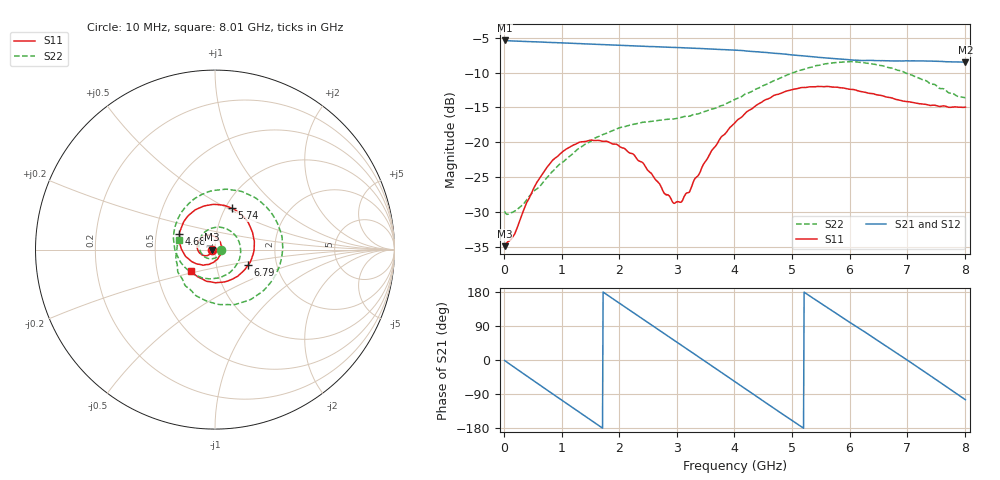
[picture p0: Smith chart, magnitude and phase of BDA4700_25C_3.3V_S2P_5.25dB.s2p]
!Agilent Technologies,E5071B,MY42404982,A.09.10
!Date: Mon Oct 20 18:05:11 2025
!Data & Calibration Information:
!Freq	S11:SOLT2(ON)	S21:SOLT2(ON)	S12:SOLT2(ON)	S22:SOLT2(ON)
# Hz S RI R 50
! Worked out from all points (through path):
!   801 points, 10 MHz to 8.01 GHz, reference 50 ohm
!   highest |S21| = -5.37 dB at 10 MHz (marker M1); lowest = -8.5 dB at 8.01 GHz (marker M2)
!   group delay of S21, straight-line fit = 285 ps
!   lowest |S11| = -34.9 dB at 10 MHz (marker M3), VSWR 1.04, Z = 48.2 - j0.11 ohm
!   |S11| at or under -10 dB: start of sweep to end of sweep
!   |S22| runs from -30.4 to -8.4 dB; largest |S21 - S12| = 0.0063
!   S11 on the Smith chart (normalised r, x): 10 MHz: 0.96, -0.00; 4.68 GHz: 0.66, +0.12; 5.74 GHz: 1.07, +0.53; 6.79 GHz: 1.43, -0.26; 8.01 GHz: 0.74, -0.18
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1e7  -0.0179 -0.00113  0.5387 -0.0118  0.5388 -0.0121  0.0317 -0.00258
3.3e8  -0.0239 -0.0207  0.4328 -0.307  0.4325 -0.3072  0.0222 -0.028
7.1e8  -0.0526 -0.0343  0.1322 -0.5064  0.1321 -0.5064  -0.0163 -0.0511
1.02e9  -0.0831 -0.0214  -0.1581 -0.4922  -0.1584 -0.4926  -0.0622 -0.0363
1.35e9  -0.0998 0.0138  -0.4038 -0.3121  -0.4041 -0.3124  -0.0901 0.0229
1.93e9  -0.06 0.0762  -0.4601 0.1917  -0.4603 0.1914  -0.00232 0.123
2.32e9  -0.0081 0.0741  -0.224 0.4365  -0.224 0.4368  0.1007 0.0921
2.68e9  0.0292 0.0422  0.0838 0.4775  0.0832 0.4774  0.1433 -0.00884
3.05e9  0.0351 -0.0118  0.3569 0.3184  0.3538 0.3208  0.0964 -0.1144
3.36e9  0.0103 -0.0561  0.4653 0.0819  0.4659 0.0821  0.00735 -0.1593
3.67e9  -0.0425 -0.0831  0.432 -0.1749  0.432 -0.1764  -0.0969 -0.1466
4.01e9  -0.1175 -0.0729  0.2476 -0.3864  0.2483 -0.3856  -0.19 -0.0718
4.34e9  -0.1783 -0.0129  -0.0116 -0.4479  -0.0116 -0.4486  -0.2307 0.0516
4.68e9  -0.1984 0.0869  -0.2609 -0.3491  -0.2599 -0.3507  -0.1949 0.1957
5.02e9  -0.1509 0.1866  -0.4013 -0.134  -0.4026 -0.1346  -0.0706 0.3087
5.35e9  -0.0504 0.2451  -0.3971 0.1086  -0.3976 0.1062  0.1047 0.331
5.74e9  0.0919 0.2313  -0.2322 0.3242  -0.2315 0.3239  0.2983 0.2237
6.18e9  0.2004 0.117  0.0535 0.3835  0.0577 0.3842  0.374 -0.0248
6.68e9  0.2025 -0.0543  0.3259 0.2038  0.3269 0.2029  0.2224 -0.2624
6.79e9  0.1845 -0.0863  0.3581 0.1377  0.3593 0.1355  0.1688 -0.2884
7.3e9  0.0544 -0.1798  0.3285 -0.1981  0.3283 -0.1986  -0.0982 -0.2615
8.01e9  -0.1344 -0.1179  -0.0964 -0.3631  -0.0955 -0.3637  -0.2011 0.0557
